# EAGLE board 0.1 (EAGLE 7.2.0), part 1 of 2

Size 160 x 100 mm. Coordinates in mm from the lower left corner, seen from the top.
Outline: 0,0 160,0 160,100 0,100 0,0
Copper layers (1*16): Top 0.035mm / dielectric 1.5mm / Bottom 0.035mm
Design rules "default": minimum track width 10mil, minimum drill 24mil, track to track 8mil, track to pad 8mil, pad to pad 8mil, via to via 8mil, smd to smd 8mil, copper to edge 40mil, drill to drill 8mil, minimum pad ring 10mil, minimum via ring 8mil, stop-mask expansion 4mil, vias tented up to drill 0mil, thermal gap 10mil

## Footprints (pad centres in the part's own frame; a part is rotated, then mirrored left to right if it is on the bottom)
0207/10 = drill 0.813 octagon: 1 -5.08,0; 2 5.08,0
C050-025X075 = drill 0.813 octagon: 1 -2.54,0; 2 2.54,0
E5-10,5 = drill 1.016 pad 2.54: + -2.54,0 | drill 1.016 pad 2.54 octagon: - 2.54,0
E2,5-5 = drill 0.813 pad 1.6: + -1.27,0 | drill 0.813 pad 1.6 octagon: - 1.27,0
E2,5-6 = drill 0.813 pad 1.6: + -1.27,0 | drill 0.813 pad 1.6 octagon: - 1.27,0
C050-035X075 = drill 0.813 octagon: 1 -2.54,0; 2 2.54,0
DIL20 = drill 0.813 long: 1 -11.43,-3.81; 2 -8.89,-3.81; 3 -6.35,-3.81; 4 -3.81,-3.81; 5 -1.27,-3.81; 6 1.27,-3.81; 7 3.81,-3.81; 8 6.35,-3.81; 9 8.89,-3.81; 10 11.43,-3.81; 11 11.43,3.81; 12 8.89,3.81; 13 6.35,3.81; 14 3.81,3.81; 15 1.27,3.81; 16 -1.27,3.81; 17 -3.81,3.81; 18 -6.35,3.81; 19 -8.89,3.81; 20 -11.43,3.81
DIL14 = drill 0.813 long: 1 -7.62,-3.81; 2 -5.08,-3.81; 3 -2.54,-3.81; 4 0,-3.81; 5 2.54,-3.81; 6 5.08,-3.81; 7 7.62,-3.81; 8 7.62,3.81; 9 5.08,3.81; 10 2.54,3.81; 11 0,3.81; 12 -2.54,3.81; 13 -5.08,3.81; 14 -7.62,3.81
DIL08 = drill 0.813 long: 1 -3.81,-3.81; 2 -1.27,-3.81; 3 1.27,-3.81; 4 3.81,-3.81; 5 3.81,3.81; 6 1.27,3.81; 7 -1.27,3.81; 8 -3.81,3.81
DIL24-3 = drill 0.813 long: 1 -13.97,-3.81; 2 -11.43,-3.81; 3 -8.89,-3.81; 4 -6.35,-3.81; 5 -3.81,-3.81; 6 -1.27,-3.81; 7 1.27,-3.81; 8 3.81,-3.81; 9 6.35,-3.81; 10 8.89,-3.81; 11 11.43,-3.81; 12 13.97,-3.81; 13 13.97,3.81; 14 11.43,3.81; 15 8.89,3.81; 16 6.35,3.81; 17 3.81,3.81; 18 1.27,3.81; 19 -1.27,3.81; 20 -3.81,3.81; 21 -6.35,3.81; 22 -8.89,3.81; 23 -11.43,3.81; 24 -13.97,3.81
PICOFUSE = drill 0.813 long: 1 -5.08,0; 2 5.08,0
JP1 = drill 0.914 long: 1 0,-1.27; 2 0,1.27
G2RA = drill 1.321 long: 1 -3.81,-3.683; 2 -3.81,3.81; P 16.18,3.81; S 19.685,-3.683
SFH480 = drill 0.813 long: A 1.27,0; K -1.27,0
P1-20Y = drill 2.007 pad 2.54 long: TP 0,0
TO220H = drill 1.118 long: 1 -2.54,-10.16; 2 0,-10.16; 3 2.54,-10.16 | hole 3.302: 0,4.826
RTRIM64Y = drill 0.61: 1 0,-2.54; 2 -2.54,0; 3 0,2.54
HC49TL-H = drill 0.813: 1 -2.413,-7.62; 2 2.413,-7.62; 3 0,7.874
0617/17 = drill 1.016 octagon: 1 -8.89,0; 2 8.89,0
TO92-CBE = drill 0.813 long: B 0,0; C -2.54,0; E 2.54,0
DO41-10 = drill 1.118: A 5.08,0; C -5.08,0
SOD81 = drill 1.118 long: A 5.08,0; C -5.08,0
DO15-12 = drill 1.118 long: A 6.35,0; C -6.35,0
DO35-10 = drill 0.813 long: A 5.08,0; C -5.08,0
S18P = drill 1.016 long: 1 21.25,0; 2 18.75,0; 3 16.25,0; 4 13.75,0; 5 11.25,0; 6 8.75,0; 7 6.25,0; 8 3.75,0; 9 1.25,0; 10 -1.25,0; 11 -3.75,0; 12 -6.25,0; 13 -8.75,0; 14 -11.25,0; 15 -13.75,0; 16 -16.24,0; 17 -18.755,0; 18 -21.244,0
AK300/2 = drill 1.321 long: 1 -2.515,0; 2 2.489,0
S06P = drill 1.016 long: 1 6.25,0; 2 3.75,0; 3 1.25,0; 4 -1.25,0; 5 -3.75,0; 6 -6.25,0
5566-12 = drill 1.4 square: 1 10.5,-2.75; 2 6.3,-2.75; 3 2.1,-2.75; 4 -2.1,-2.75; 5 -6.3,-2.75; 6 -10.5,-2.75; 7 10.5,2.75; 8 6.3,2.75; 9 2.1,2.75; 10 -2.1,2.75; 11 -6.3,2.75; 12 -10.5,2.75 | hole 3: 15.2,2.29; -15.2,2.29

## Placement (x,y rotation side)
75-  [0207/10]  not placed on the board
C1  [C050-025X075]  0,0 0 top
C1-  [E5-10,5]  0,0 0 top
C2  [E2,5-5]  not placed on the board
C2-  [E5-10,5]  0,0 0 top
C3  [C050-025X075]  not placed on the board
C3-  [E5-10,5]  0,0 0 top
C4  [C050-025X075]  not placed on the board
C4-  [E2,5-6]  0,0 0 top
C5  [C050-025X075]  0,0 0 top
C5-  [E5-10,5]  0,0 0 top
C6  [E2,5-5]  0,0 0 top
C6-  [E5-10,5]  0,0 0 top
C7  [E2,5-6]  0,0 0 top
C8-  [E5-10,5]  0,0 0 top
C9-  330nF  [C050-035X075]  0,0 0 top
C10  [E2,5-5]  0,0 0 top
C10-  330nF  [C050-035X075]  0,0 0 top
C11  [E2,5-5]  0,0 0 top
C11-  [C050-035X075]  not placed on the board
C12  [E2,5-5]  0,0 0 top
C12-  330nF  [C050-035X075]  0,0 0 top
C13  330nF  [C050-035X075]  0,0 0 top
C13-  330nF  [C050-035X075]  0,0 0 top
C14  330nF  [C050-035X075]  0,0 0 top
C14-  [C050-025X075]  not placed on the board
C15  [C050-025X075]  0,0 0 top
C16  [C050-025X075]  0,0 0 top
C16-  [C050-025X075]  0,0 0 top
C17  [C050-025X075]  0,0 0 top
C18  [C050-025X075]  0,0 0 top
C19  [C050-025X075]  0,0 0 top
C19-  [E2,5-5]  0,0 0 top
C20  330nF  [C050-035X075]  0,0 0 top
C22-  [C050-025X075]  0,0 0 top
C23  [C050-025X075]  not placed on the board
C24-  [E2,5-5]  not placed on the board
C25  [E2,5-5]  not placed on the board
C25-  [C050-025X075]  0,0 0 top
C26  330nF  [C050-035X075]  not placed on the board
C26-  [C050-025X075]  not placed on the board
C27-  [C050-025X075]  0,0 0 top
C28  [C050-035X075]  not placed on the board
C28-  [E2,5-5]  not placed on the board
C29  [E2,5-6]  0,0 0 top
C29-  [E2,5-5]  not placed on the board
C30  330nF  [C050-025X075]  not placed on the board
C30-  330nF  [C050-035X075]  not placed on the board
C31  [E2,5-6]  0,0 0 top
C31-  330nF  [C050-035X075]  not placed on the board
C32  [C050-025X075]  0,0 0 top
C33  [E2,5-6]  0,0 0 top
C34  330nF  [C050-035X075]  0,0 0 top
C35  [C050-025X075]  not placed on the board
C36  [C050-025X075]  not placed on the board
C37  [C050-035X075]  not placed on the board
C40  [C050-025X075]  not placed on the board
C41  [C050-025X075]  not placed on the board
C41-  330nF  [C050-035X075]  0,0 0 top
C42  [E2,5-5]  not placed on the board
C43  [E2,5-5]  not placed on the board
C44  330nF  [C050-035X075]  0,0 0 top
C44-  330nF  [C050-035X075]  0,0 0 top
C49  [C050-025X075]  not placed on the board
C50  [C050-025X075]  not placed on the board
C51  [C050-025X075]  not placed on the board
C52  330nF  [C050-035X075]  not placed on the board
C52-  [C050-025X075]  0,0 0 top
C53  330nF  [C050-035X075]  not placed on the board
C54  [E2,5-5]  not placed on the board
C55  [E2,5-5]  not placed on the board
C56  [C050-025X075]  0,0 0 top
C57  [C050-025X075]  0,0 0 top
C57-  [C050-025X075]  not placed on the board
C58  330nF  [C050-035X075]  0,0 0 top
C59  330nF  [C050-035X075]  not placed on the board
C60  330nF  [C050-035X075]  0,0 0 top
C60-  [C050-035X075]  0,0 0 top
C61  [C050-025X075]  0,0 0 top
C62  [C050-025X075]  0,0 0 top
C63  330nF  [C050-035X075]  not placed on the board
C65  [E2,5-5]  not placed on the board
C66  [E2,5-5]  not placed on the board
C69  [C050-025X075]  not placed on the board
C70  [C050-025X075]  not placed on the board
C71  [C050-025X075]  not placed on the board
C72  [C050-025X075]  not placed on the board
C73  [E2,5-5]  not placed on the board
C74  [E2,5-5]  not placed on the board
C76  [C050-025X075]  not placed on the board
C77  [C050-025X075]  not placed on the board
C79  [C050-025X075]  not placed on the board
C81  [C050-025X075]  not placed on the board
C82  330nF  [C050-025X075]  not placed on the board
C83  [C050-025X075]  not placed on the board
C84  [C050-025X075]  not placed on the board
C85  [C050-025X075]  not placed on the board
C86  [C050-025X075]  not placed on the board
C87  [C050-025X075]  not placed on the board
C88  [C050-025X075]  not placed on the board
C91  [C050-025X075]  not placed on the board
C92  [C050-025X075]  not placed on the board
C93  10nF  [C050-025X075]  not placed on the board
C94  [C050-025X075]  0,0 0 top
C97  [C050-025X075]  not placed on the board
C98  330nF  [C050-025X075]  not placed on the board
C98-  10nF  [C050-025X075]  not placed on the board
C99  [C050-025X075]  not placed on the board
C103-  [E2,5-5]  not placed on the board
C104  [E2,5-5]  not placed on the board
C105  [C050-025X075]  not placed on the board
C106  [C050-025X075]  not placed on the board
C106-  330nF  [C050-035X075]  not placed on the board
C107-  [C050-025X075]  not placed on the board
C109  330nF  [C050-035X075]  not placed on the board
C111  330nF  [C050-035X075]  not placed on the board
C112  330nF  [C050-035X075]  not placed on the board
C113  330nF  [C050-035X075]  not placed on the board
C114  330nF  [C050-035X075]  not placed on the board
C115  330nF  [C050-035X075]  not placed on the board
C116  330nF  [C050-035X075]  not placed on the board
C117  330nF  [C050-035X075]  not placed on the board
C118  330nF  [C050-025X075]  not placed on the board
C119-1  [C050-035X075]  0,0 0 top
C120  330nF  [C050-025X075]  not placed on the board
C123  [C050-025X075]  not placed on the board
C126  330nF  [C050-025X075]  not placed on the board
C128-  [C050-025X075]  0,0 0 top
C129-  [C050-025X075]  0,0 0 top
C130  [C050-025X075]  not placed on the board
D1-  [DIL20]  not placed on the board
D2-  [DIL14]  not placed on the board
D3-  [DIL14]  not placed on the board
D5-1  [DIL14]  not placed on the board
D6  [DIL08]  0,0 0 top
D7  [DIL08]  0,0 0 top
D8-AC-FREQ-VOLTAGE/3.12V-FIXED-VOLTAGE  [DIL08]  0,0 0 top
D9-N12/1-TRIANGE-INTEGRATOR-POS/NEG-BIAS-CURR-SWITCH  [DIL08]  0,0 0 top
D10-AC-BAL-SWITCH  [DIL08]  0,0 0 top
D12-2  [DIL08]  not placed on the board
D14  [DIL08]  0,0 0 top
D15  [DIL14]  0,0 0 top
D16  [DIL14]  0,0 0 top
D17-2  [DIL20]  not placed on the board
D18  [DIL24-3]  not placed on the board
F11  FUSEPICOFUSE  [PICOFUSE]  0,0 0 top
IC1  [DIL14]  0,0 0 top
IC6  [DIL14]  0,0 0 top
IC13-AC-MOSFET-DRIVER-OPEN-COLLECTOR  [DIL14]  0,0 0 top
IC16  [DIL14]  0,0 0 top
JP1  [JP1]  not placed on the board
JP2  [JP1]  not placed on the board
JP3  [JP1]  not placed on the board
JP7  [JP1]  not placed on the board
JP8  [JP1]  not placed on the board
JP10  [JP1]  not placed on the board
JP11  [JP1]  not placed on the board
JP12  [JP1]  not placed on the board
JP13  [JP1]  not placed on the board
JP14  [JP1]  not placed on the board
JP15  [JP1]  not placed on the board
JP17  [JP1]  not placed on the board
K1  G2RA  [G2RA]  not placed on the board
LED1/+5V  [SFH480]  not placed on the board
LED1/+15V  [SFH480]  not placed on the board
LED1/-15V  [SFH480]  not placed on the board
LED1/ACDC  [SFH480]  not placed on the board
LED1/RGLSPR  [SFH480]  not placed on the board
LED1/STRSTP  [SFH480]  not placed on the board
LED2/IGRO  [SFH480]  not placed on the board
LED2/IPRUE  [SFH480]  not placed on the board
LED2/POLARITY  [SFH480]  not placed on the board
LED2/PRUE  [SFH480]  not placed on the board
LED2/PRUN  [SFH480]  not placed on the board
LED2/SEKUE  [SFH480]  not placed on the board
LED2/STOER  [SFH480]  not placed on the board
LED2/TEMP  [SFH480]  not placed on the board
M1  TPPAD1-20Y  [P1-20Y]  0,0 0 top
M2  TPPAD1-20Y  [P1-20Y]  0,0 0 top
M3  TPPAD1-20Y  [P1-20Y]  0,0 0 top
M4  TPPAD1-20Y  [P1-20Y]  0,0 0 top
M5  TPPAD1-20Y  [P1-20Y]  0,0 0 top
M6  TPPAD1-20Y  [P1-20Y]  0,0 0 top
M7  TPPAD1-20Y  [P1-20Y]  0,0 0 top
M8  TPPAD1-20Y  [P1-20Y]  0,0 0 top
M10  TPPAD1-20Y  [P1-20Y]  not placed on the board
M11  TPPAD1-20Y  [P1-20Y]  0,0 0 top
M13  TPPAD1-20Y  [P1-20Y]  not placed on the board
M15  TPPAD1-20Y  [P1-20Y]  not placed on the board
M18  TPPAD1-20Y  [P1-20Y]  not placed on the board
M19  TPPAD1-20Y  [P1-20Y]  not placed on the board
M20  TPPAD1-20Y  [P1-20Y]  not placed on the board
M21  TPPAD1-20Y  [P1-20Y]  not placed on the board
M22-AC-BALANCED-AC-FREQ  TPPAD1-20Y  [P1-20Y]  not placed on the board
MINUSPOL  [SFH480]  not placed on the board
N1  7815-PosReg  [TO220H]  not placed on the board
N2  7805-PosReg  [TO220H]  not placed on the board
N3  7915-NegReg  [TO220H]  not placed on the board
N5-TEMP-SENSOR  [DIL08]  not placed on the board
N6  [DIL08]  not placed on the board
N7-?-?-?-TRIANGLE-INTO-VARIABLE-WIDTH-PULSE-(AC-BAL)  [DIL14]  0,0 0 top
N8  [DIL14]  0,0 0 top
N9  [DIL14]  0,0 0 top
N10  [DIL14]  0,0 0 top
N11/FREQ/FREQ/BAL/FREQ  [DIL14]  0,0 0 top
N12  [DIL14]  0,0 0 top
P1  [RTRIM64Y]  not placed on the board
P3  [RTRIM64Y]  not placed on the board
P4  [RTRIM64Y]  not placed on the board
P5  [RTRIM64Y]  not placed on the board
P7-I-MIN  [RTRIM64Y]  not placed on the board
P8  [RTRIM64Y]  not placed on the board
P8-AC-FREQ-MIN  [RTRIM64Y]  not placed on the board
P10-AC-FREQ  [RTRIM64Y]  not placed on the board
P11  [RTRIM64Y]  not placed on the board
P12-AC-BAL  1k  [RTRIM64Y]  not placed on the board
PLUSPOL  [SFH480]  not placed on the board
Q1  [HC49TL-H]  not placed on the board
R1  [0207/10]  not placed on the board
R2  [0207/10]  not placed on the board
R2-  [0207/10]  not placed on the board
R3  [0207/10]  not placed on the board
R4  [0207/10]  0,0 0 top
R4-  22k  [0207/10]  not placed on the board
R5  [0207/10]  0,0 0 top
R5-  [0207/10]  not placed on the board
R6-  [0207/10]  0,0 0 top
R7-  [0207/10]  not placed on the board
R9-  [0207/10]  not placed on the board
R10-  [0207/10]  not placed on the board
R14-  [0207/10]  0,0 0 top
R15-  [0207/10]  0,0 0 top
R16-  [0207/10]  0,0 0 top
R17-  [0207/10]  not placed on the board
R18-  [0207/10]  not placed on the board
R19  [RTRIM64Y]  not placed on the board
R19-  [0207/10]  not placed on the board
R21-  [0207/10]  0,0 0 top
R22-  [0207/10]  0,0 0 top
R23-  [0207/10]  0,0 0 top
R24-  [0207/10]  0,0 0 top
R26-  [0207/10]  not placed on the board
R28  [0207/10]  not placed on the board
R28-  [0207/10]  0,0 0 top
R29  1k  [0207/10]  0,0 0 top
R30  [0207/10]  0,0 0 top
R33-  [0207/10]  0,0 0 top
R34  [0207/10]  0,0 0 top
R35-  [0207/10]  not placed on the board
R37  [0207/10]  not placed on the board
R37-  [0207/10]  not placed on the board
R38  [0207/10]  not placed on the board
R38-  [0207/10]  0,0 0 top
R39  [0207/10]  not placed on the board
R39-  100  [0207/10]  0,0 0 top
R40  [0207/10]  not placed on the board
R43  [0207/10]  0,0 0 top
R44  [0207/10]  0,0 0 top
R44-  [0207/10]  0,0 0 top
R45  [0207/10]  0,0 0 top
R46  [0207/10]  0,0 0 top
R46-  [0207/10]  0,0 0 top
R49  [0207/10]  0,0 0 top
R50  [0207/10]  0,0 0 top
R50-  22k  [0207/10]  0,0 0 top
R51  [0207/10]  0,0 0 top
R51-  [0207/10]  not placed on the board
R52  [0207/10]  0,0 0 top
R52-  [0207/10]  not placed on the board
R53  [0207/10]  0,0 0 top
R53-  [0207/10]  not placed on the board
R54  [0207/10]  0,0 0 top
R54-  [0207/10]  not placed on the board
R55  [0207/10]  not placed on the board
R56  [0207/10]  not placed on the board
R56-  [0207/10]  0,0 0 top
R57-  [0207/10]  0,0 0 top
R58  [0207/10]  not placed on the board
R59  1k  [0207/10]  0,0 0 top
R60  1k  [0207/10]  0,0 0 top
R60-FAT  [0617/17]  not placed on the board
R61-FAT  [0617/17]  not placed on the board
R61-PULLDOWN-GND  10k  [0207/10]  0,0 0 top
R62  22k  [0207/10]  0,0 0 top
R62-FAT  [0617/17]  0,0 0 top
R63  1k  [0207/10]  0,0 0 top
R63-FAT  [0617/17]  0,0 0 top
R64  [0207/10]  not placed on the board
R65-  470  [0207/10]  not placed on the board
R65-+5V-PULLUP  [0207/10]  0,0 0 top
R66  [0207/10]  0,0 0 top
R66-  3,3k  [0207/10]  not placed on the board
R67  [0207/10]  0,0 0 top
R68  [0207/10]  0,0 0 top
R68-  3,3k  [0207/10]  not placed on the board
R69  [0207/10]  0,0 0 top
R69-  [0207/10]  0,0 0 top
R70  [0207/10]  0,0 0 top
R71  4.7k  [0207/10]  not placed on the board
R71-  [0207/10]  0,0 0 top
R72  [0207/10]  not placed on the board
R72-  [0207/10]  0,0 0 top
R73  [0207/10]  not placed on the board
R73-  [0207/10]  not placed on the board
R74  [0207/10]  not placed on the board
R74-  [0207/10]  not placed on the board
R75  [0207/10]  0,0 0 top
R76  [0207/10]  0,0 0 top
R77  [0207/10]  0,0 0 top
R78  [0207/10]  0,0 0 top
R79  [0207/10]  0,0 0 top
R80  [0207/10]  0,0 0 top
R81-  [0207/10]  0,0 0 top
R82-FAT  [0617/17]  0,0 0 top
R83  [0207/10]  0,0 0 top
R83-FAT  [0617/17]  0,0 0 top
R84  [0207/10]  0,0 0 top
R84-FAT  [0617/17]  0,0 0 top
R85-FAT  [0617/17]  0,0 0 top
R86-  [0207/10]  not placed on the board
R87  4.7k  [0207/10]  not placed on the board
R87-  [0207/10]  not placed on the board
R88  22k  [0207/10]  not placed on the board
R89  [0207/10]  not placed on the board
R90-  [0207/10]  not placed on the board
R91  [0207/10]  not placed on the board
R92-  [0207/10]  not placed on the board
R93  [0207/10]  not placed on the board
R94  [0207/10]  not placed on the board
R95  [0207/10]  not placed on the board
R95-  [0207/10]  not placed on the board
R96  [0207/10]  not placed on the board
R96-  [0207/10]  not placed on the board
R97  [0207/10]  not placed on the board
R97-  22k  [0207/10]  not placed on the board
R98  22k  [0207/10]  not placed on the board
R98-  22k  [0207/10]  not placed on the board
R99  [0207/10]  not placed on the board
R99-  22k  [0207/10]  not placed on the board
R100  [0207/10]  not placed on the board
R100-  [0207/10]  not placed on the board
R101  [0207/10]  not placed on the board
R102  [0207/10]  not placed on the board
R102-  [0207/10]  not placed on the board
R103  [0207/10]  not placed on the board
R103-  [0207/10]  not placed on the board
R104  [0207/10]  not placed on the board
R104-  [0207/10]  not placed on the board
R105  22k  [0207/10]  not placed on the board
R105-  [0207/10]  not placed on the board
R106  22k  [0207/10]  not placed on the board
R107  [0207/10]  not placed on the board
R108  22k  [0207/10]  not placed on the board
R108-  [0207/10]  not placed on the board
R109  [0207/10]  not placed on the board
R110  [0207/10]  not placed on the board
R110-  [0207/10]  not placed on the board
R111  [0207/10]  not placed on the board
R112  [0207/10]  not placed on the board
R113  22k  [0207/10]  not placed on the board
R113-  [0207/10]  not placed on the board
R114  [0207/10]  not placed on the board
R116  [0207/10]  not placed on the board
R117-FUSE+15V  FUSEPICOFUSE  [PICOFUSE]  0,0 0 top
R118-FUSE  FUSEPICOFUSE  [PICOFUSE]  0,0 0 top
R119  [0207/10]  not placed on the board
R119-FUSE-  FUSEPICOFUSE  [PICOFUSE]  0,0 0 top
R120  [0207/10]  not placed on the board
R121  [0207/10]  not placed on the board
R122  [0207/10]  not placed on the board
R123  [0207/10]  not placed on the board
R123-  [0207/10]  not placed on the board
R124-  [0207/10]  not placed on the board
R125  [0207/10]  not placed on the board
R127  [0207/10]  not placed on the board
R128  4.7k  [0207/10]  not placed on the board
R129  [0207/10]  not placed on the board
R135-  [0207/10]  not placed on the board
R136-  [0207/10]  not placed on the board
R137-  [0207/10]  not placed on the board
R138-  [0207/10]  not placed on the board
R139-  [0207/10]  not placed on the board
R141-  [0207/10]  not placed on the board
R142  [0207/10]  not placed on the board
R143  [0207/10]  not placed on the board
R144  [0207/10]  not placed on the board
R145  [0207/10]  not placed on the board
R147  [0207/10]  not placed on the board
R148-  [0207/10]  not placed on the board
R149-  [0207/10]  not placed on the board
R150  10k  [0207/10]  0,0 0 top
R150-  [0207/10]  not placed on the board
R151  [0207/10]  not placed on the board
R151-  [0207/10]  not placed on the board
R153-  [0207/10]  0,0 0 top
R154-  [0207/10]  not placed on the board
R155  [0207/10]  not placed on the board
R155-  22k  [0207/10]  not placed on the board
R156  470  [0207/10]  not placed on the board
R156-  [0207/10]  not placed on the board
R157  470  [0207/10]  not placed on the board
R157-  [0207/10]  0,0 0 top
R159  22k  [0207/10]  0,0 0 top
R160  [0207/10]  0,0 0 top
R161  [0207/10]  0,0 0 top
R162  [0207/10]  0,0 0 top
R164-FUSE  FUSEPICOFUSE  [PICOFUSE]  0,0 0 top
R165  [0207/10]  0,0 0 top
R166-  [0207/10]  not placed on the board
R167-  [0207/10]  not placed on the board
R168-  [0207/10]  not placed on the board
R170  [0207/10]  not placed on the board
R171  [0207/10]  not placed on the board
R172  [0207/10]  not placed on the board
R173  22k  [0207/10]  not placed on the board
R174  [0207/10]  not placed on the board
R175  [0207/10]  not placed on the board
R175-  [0207/10]  not placed on the board
R176  [0207/10]  not placed on the board
R177  22k  [0207/10]  not placed on the board
R178  22k  [0207/10]  not placed on the board
R179  [0207/10]  not placed on the board
R180  [0207/10]  not placed on the board
R181  [0207/10]  not placed on the board
R181-  1k  [0207/10]  not placed on the board
R182  [0207/10]  not placed on the board
R183  [0207/10]  not placed on the board
R183-  4.7k  [0207/10]  not placed on the board
R184  [0207/10]  not placed on the board
R184-  4.7k  [0207/10]  not placed on the board
R185  [0207/10]  not placed on the board
R185-  4.7k  [0207/10]  not placed on the board
R186-  4.7k  [0207/10]  not placed on the board
R187-  [0207/10]  not placed on the board
R188  [0207/10]  not placed on the board
R189  [0207/10]  not placed on the board
R190  22k  [0207/10]  not placed on the board
R191  22k  [0207/10]  not placed on the board
R192  22k  [0207/10]  not placed on the board
R193-FEEDBK-2  3,3k  [0207/10]  not placed on the board
R194-FEEDBK-1  4.7k  [0207/10]  not placed on the board
R195  [0207/10]  not placed on the board
R196  [0207/10]  not placed on the board
R197  [0207/10]  not placed on the board
R199  [0207/10]  not placed on the board
R200  [0207/10]  not placed on the board
R201  22k  [0207/10]  not placed on the board
R202  [0207/10]  not placed on the board
R203  22k  [0207/10]  not placed on the board
R208  [0207/10]  not placed on the board
R209  [0207/10]  not placed on the board
R211  22k  [0207/10]  not placed on the board
R212  22k  [0207/10]  not placed on the board
R213-5V-PULLUP  22k  [0207/10]  not placed on the board
R214  22k  [0207/10]  not placed on the board
R220  [0207/10]  not placed on the board
R222  [0207/10]  not placed on the board
R223  22k  [0207/10]  not placed on the board
R226  [0207/10]  not placed on the board
R227  [0207/10]  not placed on the board
R228  4.7k  [0207/10]  not placed on the board
R229  [0207/10]  0,0 0 top
R230  4.7k  [0207/10]  not placed on the board
R232  4.7k  [0207/10]  not placed on the board
R234  4.7k  [0207/10]  not placed on the board
R235  [0207/10]  not placed on the board
R236  [0207/10]  not placed on the board
R237  4.7k  [0207/10]  not placed on the board
R249  [0207/10]  not placed on the board
R250  [0207/10]  not placed on the board
R251  [0207/10]  not placed on the board
R253  [0207/10]  not placed on the board
R254  [0207/10]  not placed on the board
R255  [0207/10]  not placed on the board
R256  [0207/10]  not placed on the board
R257  [0207/10]  not placed on the board
R259  10k  [0207/10]  not placed on the board
R260  10k  [0207/10]  not placed on the board
R261  10k  [0207/10]  not placed on the board
R262  4.7k  [0207/10]  not placed on the board
R263-FUSE  FUSEPICOFUSE  [PICOFUSE]  0,0 0 top
R263-FUSE1  FUSEPICOFUSE  [PICOFUSE]  0,0 0 top
R263-FUSE2+15V  FUSEPICOFUSE  [PICOFUSE]  0,0 0 top
R264  [0207/10]  0,0 0 top
R265  [0207/10]  not placed on the board
R268  [0207/10]  not placed on the board
R269  [0207/10]  not placed on the board
R270  [0207/10]  not placed on the board
R272-FUSE  FUSEPICOFUSE  [PICOFUSE]  0,0 0 top
R273-FUSE  FUSEPICOFUSE  [PICOFUSE]  0,0 0 top
R274-FUSE  FUSEPICOFUSE  [PICOFUSE]  0,0 0 top
R275-FUSE  FUSEPICOFUSE  [PICOFUSE]  0,0 0 top
R276-FUSE  FUSEPICOFUSE  [PICOFUSE]  0,0 0 top
R277  [0207/10]  0,0 0 top
R279  [0207/10]  not placed on the board
R284  [0207/10]  not placed on the board
S2  [JP1]  not placed on the board
S9  [JP1]  not placed on the board
S12-AC-WAVEFORM-SHAPE/RISETIME-1  [JP1]  not placed on the board
S12-AC-WAVEFORM-SHAPE/RISETIME-2  [JP1]  not placed on the board
S22  [JP1]  not placed on the board
S23  [JP1]  not placed on the board
T3  [TO92-CBE]  not placed on the board
T4  [TO92-CBE]  not placed on the board
T5  [TO92-CBE]  not placed on the board
T6  [TO92-CBE]  not placed on the board
T7  [TO92-CBE]  not placed on the board
T8  [TO92-CBE]  not placed on the board
T9  [TO92-CBE]  not placed on the board
T10  [TO92-CBE]  not placed on the board
T11  [TO92-CBE]  not placed on the board
T12  [TO92-CBE]  not placed on the board
T13  [TO92-CBE]  not placed on the board
T14  [TO92-CBE]  not placed on the board
T15  [TO92-CBE]  not placed on the board
T17  [TO92-CBE]  not placed on the board
T18  [TO92-CBE]  not placed on the board
T19  [TO92-CBE]  not placed on the board
T20  [TO92-CBE]  not placed on the board
T21  [TO92-CBE]  not placed on the board
T22  [TO92-CBE]  not placed on the board
T23  [TO92-CBE]  not placed on the board
T24  [TO92-CBE]  not placed on the board
T25  [TO92-CBE]  not placed on the board
TP1  TPPAD1-20Y  [P1-20Y]  0,0 0 top
V1  1N4004  [DO41-10]  0,0 0 top
V1-  1N4004  [DO41-10]  0,0 0 top
V2  BZD23  [SOD81]  0,0 0 top
V3  1N4004  [DO41-10]  0,0 0 top
V4  Diode-0.6V  [DO15-12]  0,0 0 top
V5  Diode-0.6V  [DO15-12]  0,0 0 top
V6  Diode-0.6V  [DO15-12]  0,0 0 top
V6-  BZD23  [SOD81]  0,0 0 top
V7  Diode-0.6V  [DO15-12]  0,0 0 top
V7-  BZD23  [SOD81]  0,0 0 top
V8  1N4148  [DO35-10]  0,0 0 top
V9  1N4148  [DO35-10]  0,0 0 top
V10  1N4148  [DO35-10]  not placed on the board
V11  1N4148  [DO35-10]  not placed on the board
V12  1N4148  [DO35-10]  not placed on the board
V13  1N4004  [DO41-10]  0,0 0 top
V14  Z-4.7V  [SOD81]  0,0 0 top
V17  1N4148  [DO35-10]  not placed on the board
V18  1N4148  [DO35-10]  not placed on the board
V19  1N4148  [DO35-10]  not placed on the board
V20  1N4148  [DO35-10]  not placed on the board
V21  1N4148  [DO35-10]  not placed on the board
V22  1N4148  [DO35-10]  not placed on the board
V22-NO-ZENER?  BZD23  [SOD81]  not placed on the board
V23  1N4148  [DO35-10]  not placed on the board
V24  Diode-0.6V  [DO15-12]  0,0 0 top
V25  BZD23  [SOD81]  not placed on the board
V26  1N4148  [DO35-10]  not placed on the board
V26-  1N4148  [DO35-10]  not placed on the board
V27  1N4148  [DO35-10]  not placed on the board
V28  1N4148  [DO35-10]  not placed on the board
V29  1N4148  [DO35-10]  not placed on the board
V30  1N4148  [DO35-10]  not placed on the board
V30-NOZENER  BZD23  [SOD81]  0,0 0 top
V31  1N4004  [DO41-10]  not placed on the board
V32  Diode-0.6V  [DO15-12]  0,0 0 top
V34  1N4148  [DO35-10]  not placed on the board
V35  1N4148  [DO35-10]  not placed on the board
V37  BZD23  [SOD81]  not placed on the board
V38  1N4004  [DO41-10]  not placed on the board
V39  1N4004  [DO41-10]  not placed on the board
V41  1N4148  [DO35-10]  0,0 0 top
V42  1N4148  [DO35-10]  0,0 0 top
V42-  1N4148  [DO35-10]  0,0 0 top
V43  1N4148  [DO35-10]  0,0 0 top
V43-  1N4148  [DO35-10]  0,0 0 top
V44  Diode-0.6V  [DO15-12]  0,0 0 top
V45  1N4148  [DO35-10]  not placed on the board
V46  1N4148  [DO35-10]  not placed on the board
V47  1N4148  [DO35-10]  not placed on the board
V48  1N4148  [DO35-10]  not placed on the board
V49  1N4004  [DO41-10]  0,0 0 top
V50  1N4004  [DO41-10]  0,0 0 top
V51  1N4148  [DO35-10]  not placed on the board
V52  1N4148  [DO35-10]  not placed on the board
V53  1N4148  [DO35-10]  not placed on the board
V54  1N4148  [DO35-10]  not placed on the board
V55  1N4148  [DO35-10]  not placed on the board
V55-  1N4148  [DO35-10]  not placed on the board
V56  1N4148  [DO35-10]  not placed on the board
V57  1N4148  [DO35-10]  not placed on the board
V58  1N4004  [DO41-10]  0,0 0 top
V61  Z-2.2V  [SOD81]  not placed on the board
V62  1N4148  [DO35-10]  0,0 0 top
V65  1N4148  [DO35-10]  not placed on the board
V66  1N4148  [DO35-10]  0,0 0 top
V66-NOZENER  BZD23  [SOD81]  not placed on the board
V67  1N4148  [DO35-10]  not placed on the board
V70  Diode-0.6V  [DO15-12]  not placed on the board
V72  Diode-0.6V  [DO15-12]  not placed on the board
V73  Diode-0.6V  [DO15-12]  not placed on the board
V74  Diode-0.6V  [DO15-12]  not placed on the board
V75  Diode-0.6V  [DO15-12]  not placed on the board
V76  Diode-0.6V  [DO15-12]  not placed on the board
V77  Diode-0.6V  [DO15-12]  not placed on the board
V78  Diode-0.6V  [DO15-12]  not placed on the board
V79  Diode-0.6V  [DO15-12]  not placed on the board
V80  Diode-0.6V  [DO15-12]  not placed on the board
V81  Diode-0.6V  [DO15-12]  not placed on the board
V82-NOZENER  BZD23  [SOD81]  0,0 0 top
V83  Diode-0.6V  [DO15-12]  not placed on the board
V84  1N4148  [DO35-10]  not placed on the board
V85  1N4148  [DO35-10]  not placed on the board
V91  1N4148  [DO35-10]  not placed on the board
V92  1N4148  [DO35-10]  not placed on the board
V93  1N4148  [DO35-10]  not placed on the board
V97-NOZENER  BZD23  [SOD81]  0,0 0 top
V100-NOZENER  BZD23  [SOD81]  not placed on the board
V101  1N4004  [DO41-10]  not placed on the board
V102  1N4148  [DO35-10]  not placed on the board
V102-NOZENER  BZD23  [SOD81]  0,0 0 top
V104  1N4148  [DO35-10]  not placed on the board
V105  1N4148  [DO35-10]  not placed on the board
V109-NOZENER  BZD23  [SOD81]  not placed on the board
V110  BZD23  [SOD81]  0,0 0 top
V113-NOZENER  BZD23  [SOD81]  0,0 0 top
V114  Diode-0.6V  [DO15-12]  not placed on the board
V115  1N4148  [DO35-10]  0,0 0 top
V120  1N4004  [DO41-10]  not placed on the board
V121  1N4004  [DO41-10]  not placed on the board
X1  [S18P]  not placed on the board
X2  [S18P]  not placed on the board
X3  [AK300/2]  not placed on the board
X4-  [AK300/2]  not placed on the board
X5  [S06P]  not placed on the board
X6  5566-12  [5566-12]  0,0 0 top
X7-  [AK300/2]  not placed on the board
X8  [AK300/2]  not placed on the board
X9  [S06P]  not placed on the board
X10  [S06P]  not placed on the board
X11  [S06P]  not placed on the board
X12  [AK300/2]  not placed on the board
X13  [AK300/2]  not placed on the board

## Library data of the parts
75- C1-C6 C9- C10 C10- C11 C11- C12 C12- C13 C13- C14 C14- C15 C16 C16- C17-C19 C19- C20 C22- C23 C24- C25 C25- C26 C26- C27- C28 C28- C29- C30 C30- C31- C32 C34-C37 C40 C41 C41- C42-C44 C44- C49-C52 C52- C53-C57 C57- C58-C60 C60- C61-C63 C65 C66 C69-C74 C76 C77 C79 C81-C88 C91-C94 C97 C98 C98- C99 C103- C104-C106 C106- C107- C109 C111-C118 C119-1 C120 C123 C126 C128- C129- C130 P1 P3-P5 P7-I-MIN P8 P8-AC-FREQ-MIN P10-AC-FREQ P11 P12-AC-BAL R1 R2 R2- R3 R4 R4- R5 R5- R6- R7- R9- R10- R14- R15- R16- R17- R18- R19 R19- R21- R22- R23- R24- R26- R28 R28- R29 R30 R33- R34 R35- R37 R37- R38 R38- R39 R39- R40 R43 R44 R44- R45 R46 R46- R49 R50 R50- R51 R51- R52 R52- R53 R53- R54 R54- R55 R56 R56- R57- R58-R60 R60-FAT R61-FAT R61-PULLDOWN-GND R62 R62-FAT R63 R63-FAT R64 R65- R65-+5V-PULLUP R66 R66- R67 R68 R68- R69 R69- R70 R71 R71- R72 R72- R73 R73- R74 R74- R75-R80 R81- R82-FAT R83 R83-FAT R84 R84-FAT R85-FAT R86- R87 R87- R88 R89 R90- R91 R92- R93-R95 R95- R96 R96- R97 R97- R98 R98- R99 R99- R100 R100- R101 R102 R102- R103 R103- R104 R104- R105 R105- R106-R108 R108- R109 R110 R110- R111-R113 R113- R114 R116 R119-R123 R123- R124- R125 R127-R129 R135- R136- R137- R138- R139- R141- R142-R145 R147 R148- R149- R150 R150- R151 R151- R153- R154- R155 R155- R156 R156- R157 R157- R159-R162 R165 R166- R167- R168- R170-R175 R175- R176-R181 R181- R182 R183 R183- R184 R184- R185 R185- R186- R187- R188-R192 R193-FEEDBK-2 R194-FEEDBK-1 R195-R197 R199-R203 R208 R209 R211 R212 R213-5V-PULLUP R214 R220 R222 R223 R226-R230 R232 R234-R237 R249-R251 R253-R257 R259-R262 R264 R265 R268-R270 R277 R279 R284 = resistor
C1- C2- C3- C4- C5- C6- C7 C8- C29 C31 C33 = rcl
D1- D2- D3- D5-1 D12-2 D17-2 D18 N5-TEMP-SENSOR N6 = ic-package
D6 D7 D8-AC-FREQ-VOLTAGE/3.12V-FIXED-VOLTAGE D9-N12/1-TRIANGE-INTEGRATOR-POS/NEG-BIAS-CURR-SWITCH D10-AC-BAL-SWITCH D14-D16 IC6 IC13-AC-MOSFET-DRIVER-OPEN-COLLECTOR IC16 N7-?-?-?-TRIANGLE-INTO-VARIABLE-WIDTH-PULSE-(AC-BAL) N8-N10 N11/FREQ/FREQ/BAL/FREQ N12 = 11-Wig-parts-1
F11 R117-FUSE+15V R118-FUSE R119-FUSE- R164-FUSE R263-FUSE R263-FUSE1 R263-FUSE2+15V R272-FUSE R273-FUSE R274-FUSE R275-FUSE R276-FUSE = fuse; OC_FARNELL: unknown; OC_NEWARK: unknown
IC1 = 11-Wig-parts-good
JP1-JP3 JP7 JP8 JP10-JP15 JP17 S2 S9 S12-AC-WAVEFORM-SHAPE/RISETIME-1 S12-AC-WAVEFORM-SHAPE/RISETIME-2 S22 S23 = jumper
K1 = relay; OC_FARNELL: unknown; OC_NEWARK: unknown
LED1/+5V LED1/+15V LED1/-15V LED1/ACDC LED1/RGLSPR LED1/STRSTP LED2/IGRO LED2/IPRUE LED2/POLARITY LED2/PRUE LED2/PRUN LED2/SEKUE LED2/STOER LED2/TEMP MINUSPOL PLUSPOL = led
M1-M8 M10 M11 M13 M15 M18-M21 M22-AC-BALANCED-AC-FREQ TP1 = testpad
N1-N3 = linear
Q1 = crystal; OC_FARNELL: unknown; OC_NEWARK: unknown
T3-T7 T17-T20 = transistor-neu-to92
T8-T15 T21-T25 = transistor
V1 V1- V2-V6 V6- V7 V7- V8-V14 V17-V22 V22-NO-ZENER? V23-V26 V26- V27-V30 V30-NOZENER V31 V32 V34 V35 V37-V39 V41 V42 V42- V43 V43- V44-V55 V55- V56-V58 V61 V62 V65 V66 V66-NOZENER V67 V70 V72-V81 V82-NOZENER V83-V85 V91-V93 V97-NOZENER V100-NOZENER V101 V102 V102-NOZENER V104 V105 V109-NOZENER V110 V113-NOZENER V114 V115 V120 V121 = diode
X1 X2 X5 X9-X11 = con-amp-mt; OC_FARNELL: unknown; OC_NEWARK: unknown
X3 X4- X7- X8 X12 X13 = con-ptr500; OC_FARNELL: unknown; OC_NEWARK: unknown
X6 = con-molex; OC_FARNELL: unknown; OC_NEWARK: unknown

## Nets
3.12V-FIXED: D8-AC-FREQ-VOLTAGE/3.12V-FIXED-VOLTAGE.7 R188.2 R189.1
4X-TEMPSWITCHES-COMBINED: C12.+ IC1.13 R1.2 R63.1
+5VDC: C5-.+ C6-.+ C98.1 C120.1 D15.14 D16.14 D17-2.20 D18.24 IC1.14 IC13-AC-MOSFET-DRIVER-OPEN-COLLECTOR.14 N2.3 R2-.2 R65-+5V-PULLUP.2 R212.1 R213-5V-PULLUP.1 R214.1 R253.2 R254.2 R255.2 R256.2 R279.1 R284.1
+5VDC-IN: C4-.+ N2.1 X5.3
+15VDC: C10.+ C11-.2 C28-.+ C37.1 C43.+ C54.+ C73.+ C103-.+ C104.+ D6.8 D7.3 D7.8 D8-AC-FREQ-VOLTAGE/3.12V-FIXED-VOLTAGE.3 D8-AC-FREQ-VOLTAGE/3.12V-FIXED-VOLTAGE.8 D9-N12/1-TRIANGE-INTEGRATOR-POS/NEG-BIAS-CURR-SWITCH.3 D9-N12/1-TRIANGE-INTEGRATOR-POS/NEG-BIAS-CURR-SWITCH.8 D10-AC-BAL-SWITCH.3 D10-AC-BAL-SWITCH.8 D14.8 IC6.11 JP1.1 N5-TEMP-SENSOR.7 N7-?-?-?-TRIANGLE-INTO-VARIABLE-WIDTH-PULSE-(AC-BAL).11 N8.11 N9.3 N10.3 N11/FREQ/FREQ/BAL/FREQ.11 N12.11 R40.1 R52-.1 R56.1 R93.1 R94.2 R102.2 R103-.1 R103.2 R106.1 R107.1 R108-.1 R108.1 R109.1 R112.2 R119.2 R123.2 R128.2 R166-.1 R167-.1 R182.1 R188.1 R211.1 R236.2 R249.2 R250.2 R260.1 R261.1 R263-FUSE2+15V.1 S9.2 T3.E T4.E T5.E T6.E T7.E V9.C V13.A V18.C V20.C V25.C V34.C V38.C V45.C V47.C V51.C V55-.C V55.C V58.A V105.C X1.5 X1.18 X2.2 X2.9 X6.2 X10.3 X11.3
+15VDC-IN: C1-.+ N1.1 X5.1
+15VDC-PSU: C2-.+ C3-.+ C60-.2 D12-2.8 N1.3 R117-FUSE+15V.2 R263-FUSE2+15V.2
+33VDC-IN: R50-.2 X5.6
-15VDC: C8-.- C11.- C24-.- C29-.- C55.- C66.+ C74.- D6.5 D7.5 D8-AC-FREQ-VOLTAGE/3.12V-FIXED-VOLTAGE.5 D9-N12/1-TRIANGE-INTEGRATOR-POS/NEG-BIAS-CURR-SWITCH.5 D10-AC-BAL-SWITCH.5 D14.5 IC6.7 LED1/-15V.K N3.3 N5-TEMP-SENSOR.4 N7-?-?-?-TRIANGLE-INTO-VARIABLE-WIDTH-PULSE-(AC-BAL).7 N8.7 N11/FREQ/FREQ/BAL/FREQ.7 N12.7 R116.2 R183-.1 V1.A V8.A V19.A V35.A V52.A V54.A V56.A V76.A X1.7 X2.7
-15VDC-IN: C7.- N3.2 X5.2
??12: R202.2 V61.A
AC-BAL-VOLTAGE-1: N11/FREQ/FREQ/BAL/FREQ.8 N11/FREQ/FREQ/BAL/FREQ.10 P12-AC-BAL.1
AC-BAL-VOLTAGE-2: P12-AC-BAL.2 R184-.1
AC-BAL-VOLTAGE-INVERTED: D10-AC-BAL-SWITCH.7 M18.TP N12.10 R194-FEEDBK-1.2
AC-BAL-VOLTAGE-INVERTED-TRIANGLE-TRIGGER-VOLTS: C26.1 N7-?-?-?-TRIANGLE-INTO-VARIABLE-WIDTH-PULSE-(AC-BAL).14 R100.2
AC-BALANCE/0V=20%EP: R178.2 X9.2
AC-BALANCED-AC-FREQ-PULSES-1: N7-?-?-?-TRIANGLE-INTO-VARIABLE-WIDTH-PULSE-(AC-BAL).12 R127.2 V30.C
AC-BALANCED-AC-FREQ-PULSES-2: R101.2 V30.A
AC-BALANCED-AC-FREQ-PULSES-3: JP15.2 M22-AC-BALANCED-AC-FREQ.TP R101.1 V37.C
AC-BALANCED-AC-FREQ-PULSES-4: C84.1 D18.4 JP8.1 JP15.1 R214.2
AC-FREQ-TRIANGLE-1: C41.2 M20.TP N12.3 R113.2 R208.1 R209.2
AC-FREQ-TRIANGLE-2: N7-?-?-?-TRIANGLE-INTO-VARIABLE-WIDTH-PULSE-(AC-BAL).13 R113.1 R127.1
AC-FREQ-VADJ-3: P8-AC-FREQ-MIN.2 R196.1
AC-FREQ-VOLTAGE-2: C52-.1 N8.3 R4-.1 R100-.2 S12-AC-WAVEFORM-SHAPE/RISETIME-1.2
AC-FREQ-VOLTAGE-ADJUSTED: D8-AC-FREQ-VOLTAGE/3.12V-FIXED-VOLTAGE.6 M19.TP N11/FREQ/FREQ/BAL/FREQ.4 N11/FREQ/FREQ/BAL/FREQ.6
AC-FREQ-VOLTAGE-BUFFERED: N11/FREQ/FREQ/BAL/FREQ.1 N11/FREQ/FREQ/BAL/FREQ.3 P10-AC-FREQ.3
AC-FREQ-VOLTAGE-BUFFERED-ADJ-1: P10-AC-FREQ.2 R195.2
AC-FREQ-VOLTAGE-BUFFERED-ADJ-2: C71.1 N11/FREQ/FREQ/BAL/FREQ.5 R195.1 R196.2
AC-FREQ-VOLTAGE-IN: C69.1 N11/FREQ/FREQ/BAL/FREQ.2 R177.1 V45.A V46.C
AC-FREQ-VOLTS/3.12V-FIXED: C72.2 D8-AC-FREQ-VOLTAGE/3.12V-FIXED-VOLTAGE.4 R187-.1 R190.1
AC-FREQ-VOLTS/3.12V-FIXED-2: N11/FREQ/FREQ/BAL/FREQ.14 R190.2 R191.1
AC-FREQ/0V=50HZ: R177.2 X9.1
AC-NEG-RAMP-CURRENT: D9-N12/1-TRIANGE-INTEGRATOR-POS/NEG-BIAS-CURR-SWITCH.7 R187-.2
AC-POS-RAMP-CURRENT: D9-N12/1-TRIANGE-INTEGRATOR-POS/NEG-BIAS-CURR-SWITCH.6 R197.2
AC-SQUAREWAVE-(FROM-AC-TRIANGLE)=>TRIANGLE-INTEGRATOR-BIAS-SWITCH&MINUS-LED: C42.- M21.TP MINUSPOL.A N12.4 R71.1 V10.C V11.A
AC/DC-AC=15V: R222.1 R226.2 S9.1 X9.4
ALL-TEMPSWITCHES-COMBINED: R1.1 V28.C V29.C V92.C V93.C
CHOPPER-AC-FREQ: D9-N12/1-TRIANGE-INTEGRATOR-POS/NEG-BIAS-CURR-SWITCH.2 R71.2 T5.C V12.C
D6-D7-SWITCH-ENABLE: D6.2 D7.2 D16.13 R58.1 V82-NOZENER.C V113-NOZENER.C
D6-D7-SWITCH-ENABLE-1: IC1.10 V113-NOZENER.A
D6-D7-SWITCH-ENABLE-2: IC1.4 V82-NOZENER.A
D8-SWITCH-ENABLE-(FIXED/VARIABLE-AC-FREQ): D8-AC-FREQ-VOLTAGE/3.12V-FIXED-VOLTAGE.2 M6.TP N10.2 R112.1 R202.1 V100-NOZENER.C V102-NOZENER.C
D8-SWITCH-ENABLE-(FIXED/VARIABLE-AC-FREQ)-FROM-X1/2&X3/2: C40.2 N10.5 R161.2 R162.2
GND [GND]: C1-.- C1.2 C2-.- C3-.- C4-.- C5.2 C6.- C7.+ C8-.+ C10.- C11-.1 C11.+ C12.- C13.1 C14-.2 C14.1 C15.2 C16.2 C17.2 C18.2 C19.2 C20.1 C23.1 C24-.+ C25.- C26-.1 C26.2 C27-.1 C28-.- C28.2 C29-.+ C29.+ C30-.2 C30.2 C31-.2 C31.- C33.- C34.2 C35.2 C36.1 C37.2 C40.1 C41-.1 C42.+ C43.- C44-.1 C44.2 C49.2 C50.1 C52.2 C53.2 C54.- C55.+ C56.1 C57-.2 C57.1 C59.1 C60-.1 C60.2 C61.1 C62.1 C65.+ C66.- C69.2 C70.1 C71.2 C72.1 C76.1 C77.1 C79.1 C81.2 C82.2 C83.2 C84.2 C85.2 C86.2 C87.2 C88.1 C91.1 C92.1 C93.1 C94.2 C97.1 C98-.1 C98.2 C99.1 C103-.- C104.- C105.2 C106.2 C107-.2 C111.1 C112.1 C113.1 C114.1 C115.1 C116.1 C117.1 C118.1 C120.2 C123.1 C126.1 C128-.2 C129-.2 C130.1 D1-.1 D1-.20 D2-.7 D2-.11 D2-.13 D3-.11 D5-1.7 D6.1 D7.1 D8-AC-FREQ-VOLTAGE/3.12V-FIXED-VOLTAGE.1 D9-N12/1-TRIANGE-INTEGRATOR-POS/NEG-BIAS-CURR-SWITCH.1 D10-AC-BAL-SWITCH.1 D12-2.1 D14.1 D15.7 D16.7 D17-2.10 D18.9 D18.10 D18.12 IC1.7 IC13-AC-MOSFET-DRIVER-OPEN-COLLECTOR.7 IC16.7 K1.1 LED1/+5V.K LED1/+15V.K LED1/ACDC.K LED1/RGLSPR.K LED1/STRSTP.K N1.2 N2.2 N3.1 N6.1 N6.4 N9.12 N10.12 P7-I-MIN.3 P8-AC-FREQ-MIN.3 P8.3 R3.1 R17-.1 R19.2 R19.3 R26-.1 R30.2 R39.1 R44-.1 R44.2 R51-.1 R54-.1 R58.2 R60-FAT.1 R61-FAT.1 R61-PULLDOWN-GND.1 R62-FAT.1 R63-FAT.1 R63.2 R64.2 R67.1 R70.2 R78.2 R79.2 R80.1 R83.2 R84.2 R87.2 R97-.1 R97.2 R104.2 R105.1 R110.1 R122.2 R124-.1 R137-.2 R138-.1 R139-.1 R143.1 R145.1 R149-.2 R156-.2 R157.2 R165.1 R170.1 R171.1 R172.1 R173.1 R174.1 R179.2 R180.2 R181-.1 R181.2 R183.1 R184.1 R185.1 R186-.1 R189.2 R192.2 R199.1 R251.1 R259.1 R265.2 R269.1 T8.C T9.C T10.C T11.C T12.C T13.B T14.B T15.C T17.C T18.C T19.C T20.C T25.C V1.C V5.A V12.A V13.C V24.A V32.A V37.A V39.A V44.A V46.A V50.A V57.A V70.A V72.A V73.A V74.A V75.A V76.C V77.A V78.A V79.A V80.A V81.A V83.A V85.C V104.A V114.A V120.A X1.4 X1.6 X1.11 X1.13 X1.16 X2.8 X5.4 X5.5 X6.3 X10.2 X11.2
I-PULS: R200.2 X9.3
INP-1/1-AC-SWITCH-DELAY?: C81.1 C99.2 D17-2.1 D18.1 N10.14 R65-+5V-PULLUP.1
INP-1/7-: C87.1 D17-2.2 D18.7 IC1.8 V115.A
INP-4/X-TEMP-SWITCHES: C30.1 D17-2.4 IC1.12
INP-5/X-: C105.1 D17-2.5 R253.1 V102-NOZENER.A
INP-6/X-: C106.1 D17-2.6 N9.2 R147.2 R255.1
INP-7/X-: C107-.1 D17-2.7 R256.1 V91.A
INP-8/X-: C106-.2 D17-2.8 R254.1
INP-11/X-: C109.1 D17-2.11 R2.1 R257.1 V66-NOZENER.C
INP-X/2-N5-TEMP-SENSOR-(0=>GOOD): C83.1 C119-1.1 D16.9 D18.2 M13.TP N9.14 R212.2 R277.1
INP-X/3-FIXED/VARIABLE-AC-FREQ: C82.1 D18.3 R213-5V-PULLUP.2 V100-NOZENER.A
INP-X/5-: C85.1 D18.5
INP-X/6-PLUS-MINUS-NOT-D6-D7-SWITCH-ENABLE-1: C86.1 D18.6 IC1.6 IC1.11
INP-X/15-FROM-OUTP-X/22: C98-.2 D18.14 R59.1
INP-X/23-FROM-OUTP-X/15: C93.2 D18.23 R60.1
INV-AC-FREQ-VOLTS/-3.12V-FIXED: N11/FREQ/FREQ/BAL/FREQ.12 R191.2 R197.1
N5-NEG-INP: C22-.2 N5-TEMP-SENSOR.2 R66-.1 R69-.1
N5-POS-INP: N5-TEMP-SENSOR.3 R68-.1
N5-TEMP-OUT: N5-TEMP-SENSOR.6 R39-.2 R72-.2 R155.2
N5-TEMP-OUT-2: C36.2 R110-.2 R155.1
N5-TEMP-OUT-3: N9.9 R110-.1 R270.2
N9-8-FIXED-VOLTAGE-LEVEL: C119-1.2 N9.8 R29.1 R108-.2
N10-P4/+2.411VDC-FIXED: N10.4 R102.1 R103.1 R104.1
N10-P9-FIXED-VOLTAGE-AC-SWITCH-DELAY?: N10.9 R105.2 R106.2
N10-P11-FIXED-VOLTAGE: N10.11 R108.2 R110.2
N12-P2-TO-GND: N12.2 R269.2
N12-P5-TO-GND: N12.5 R199.2
N12-P9-TO-GND: N12.9 R186-.2
N12-P13-FIXED-VOLTAGE: N12.13 R259.2 R260.2
N$1: R153-.2 R270.1
N$2: LED2/POLARITY.K R268.2
N$4: R175-.2 X2.12
N$5: N8.5 V20.A V21.C
N$6: C14.2 R75.2 R76.2
N$7: LED2/IGRO.A LED2/IPRUE.A LED2/POLARITY.A LED2/PRUE.A LED2/PRUN.A LED2/SEKUE.A LED2/STOER.A LED2/TEMP.A
N$8: D16.10 V114.C X6.6
N$9: R175-.1 V55.A V56.C
N$12: N6.8 R55.1 V49.C V121.C X12.1 X13.1
N$13: N7-?-?-?-TRIANGLE-INTO-VARIABLE-WIDTH-PULSE-(AC-BAL).10 R111.1 R141-.1
N$14: C28.1 N12.14 R261.2 R262.2 V104.C V105.A
N$17: C1.1 N7-?-?-?-TRIANGLE-INTO-VARIABLE-WIDTH-PULSE-(AC-BAL).9 R135-.1 R136-.2 R137-.1 V48.C V55-.A
N$18: T11.E V49.A V50.C X13.2
N$19: IC1.2 JP8.2
N$20: LED2/IGRO.K R228.2
N$21: JP2.2 JP3.2 R235.2
N$22: LED2/PRUN.K R232.2
N$23: LED2/SEKUE.K R237.2
N$24: LED2/TEMP.K R234.2
N$25: C32.2 V5.C X4-.2
N$26: LED1/RGLSPR.A R154-.1
N$27: MINUSPOL.K PLUSPOL.A R265.1
N$28: T12.E V120.C V121.A X12.2
N$29: D15.8 R232.1 V75.C X2.3
N$30: D15.12 JP3.1 R234.1 V77.C X2.1
N$33: C70.2 N11/FREQ/FREQ/BAL/FREQ.9 R178.1 V47.A V57.C
N$34: T7.C V7.A
N$35: R105-.2 R251.2
N$36: R193-FEEDBK-2.1 R194-FEEDBK-1.1
N$37: C15.1 N6.3 R69.2
N$38: IC6.8 IC6.10 R91.2 V18.A V19.C
N$39: C31-.1 R68.2 V41.C
N$45: N12.8 R184-.2 R185-.2 R193-FEEDBK-2.2
N$50: C52-.2 N8.1 R98-.2 R99-.2 R100-.1
N$51: M15.TP T8.E
N$52: N10.13 R68.1 R109.2
N$53: R203.2 V53.C
N$54: R141-.2 V27.A
N$55: C63.2 N8.13 R166-.2 R167-.2 R168-.2
N$56: C63.1 R95-.1 R168-.1 R257.2 V66-NOZENER.A
N$57: M1.TP N8.10 R35-.1 R151-.1
N$58: N8.8 R38.2 R150-.1
N$59: N8.12 N8.14 R176.1 V38.A V39.C
N$66: JP10.2 JP11.2 JP12.2 JP13.2 R73-.1 R90-.2
N$67: V3.A X1.17
N$70: JP7.1 N7-?-?-?-TRIANGLE-INTO-VARIABLE-WIDTH-PULSE-(AC-BAL).8 R111.2 R139-.2
N$72: D7.6 P8.2
N$74: D10-AC-BAL-SWITCH.4 R100.1
N$75: R28.1 V26.A
N$78: D1-.8 R53.1 R54.1
N$79: JP7.2 R138-.2
N$81: N7-?-?-?-TRIANGLE-INTO-VARIABLE-WIDTH-PULSE-(AC-BAL).5 R124-.2
N$84: R129.1 V26-.A V26.C V27.C
N$86: LED1/+5V.A R2-.1
N$89: N7-?-?-?-TRIANGLE-INTO-VARIABLE-WIDTH-PULSE-(AC-BAL).1 R96.1 R113-.2 R114.1 V23.A
N$90: N7-?-?-?-TRIANGLE-INTO-VARIABLE-WIDTH-PULSE-(AC-BAL).2 R97.1
N$91: C4.2 M2.TP N7-?-?-?-TRIANGLE-INTO-VARIABLE-WIDTH-PULSE-(AC-BAL).3 V23.C V26-.C
N$92: N7-?-?-?-TRIANGLE-INTO-VARIABLE-WIDTH-PULSE-(AC-BAL).4 V17.C V22.C
N$93: R98.1 V91.C
N$94: R98.2 R99.2 T9.B
N$95: D10-AC-BAL-SWITCH.6 R99.1
N$96: C3.2 R28.2 R128.1 V17.A
N$97: P8.1 R94.1
N$98: N8.6 P5.1
N$100: P4.3 R95-.2
N$101: N8.4 P4.1
N$102: D6.7 P4.2
N$103: P5.3 R96-.2
N$104: D6.6 P5.2
N$105: N8.2 R97-.2
N$106: C59.2 R155-.2 V102.A
N$111: R121.1 R122.1
N$114: R116.1 R120.1
N$116: C106-.1 C109.2
N$117: JP10.1 R174.2
N$122: N8.9 R37.2 R148-.2
N$127: C129-.1 D14.2 R38-.2 V110.A
N$130: R150-.2 R151-.2
N$133: D1-.2 R180.1
N$134: R29.2 R30.1
N$135: R19.1 R151.2
N$136: R82-FAT.1 R83-FAT.1
N$137: M4.TP R69.1 R84-FAT.1 R85-FAT.1 X1.14
N$138: R82-FAT.2 R83-FAT.2 R84-FAT.2 R85-FAT.2
N$139: S22.1 X1.9
N$140: S23.1 X1.8
N$141: T6.C V66.A
N$142: D1-.3 R55.2 R181.1
N$144: C5.1 D1-.14 P1.3
N$145: D1-.15 R84.1
N$146: C16.1 D1-.17 R79.1
N$147: IC16.8 R14-.2
N$148: D1-.19 R77.1
N$149: C18.1 D1-.13 R75.1 R76.1 R78.1
N$151: C17.1 D1-.16 R70.1 V43.C
N$152: IC16.6 R15-.2
N$153: D5-1.14 R14-.1 R15-.1
N$154: D5-1.3 R16-.1
N$155: D5-1.4 R21-.1
N$156: R28-.1 R38-.1 R56.2 T15.E V7-.C V110.C
N$157: D2-.14 D3-.14 IC16.14
N$158: R250.1 V93.A X11.1
N$160: D5-1.9 R22-.2
N$161: D5-1.10 R23-.2
N$165: R262.1 X10.6 X11.6
N$166: C22-.1 S2.1
N$167: D6.4 R98-.1
N$168: R249.1 V92.A X10.1
N$171: D15.2 JP2.1 R228.1 V72.C X2.6
N$177: N9.11 R9-.2 R19-.1 R151.1
N$182: N9.13 R9-.1
N$184: C27-.2 R39-.1
N$185: R71-.1 R72-.1
N$186: R69-.2 R71-.2
N$187: R264.2 V6.C V7.C
N$188: V4.A V6.A
N$189: D12-2.3 R150.1
N$190: R150.2 V42-.C
N$192: D12-2.7 R159.1 R160.1
N$193: R157-.2 R160.2
N$197: R161.1 V43-.C
N$198: 75-.2 JP11.1 R173.2
N$199: JP12.1 R170.2 R171.2 R172.2 R175.1
N$203: IC6.2 R86-.2
N$204: IC6.4 R5-.2 V6-.C V109-NOZENER.A
N$205: IC6.5 R37-.1
N$206: IC6.6 R4-.2 R5-.1
N$207: C25-.2 D14.4 IC6.14 R7-.2 R18-.1
N$208: C25-.1 IC6.12 R37-.2 S12-AC-WAVEFORM-SHAPE/RISETIME-2.2
N$209: IC6.9 R90-.1
N$210: IC6.13 R26-.2
N$211: R153-.1 R277.2
N$212: R7-.1 V109-NOZENER.C
N$213: R157-.1 T7.B V42-.A
N$214: C62.2 D12-2.2 D12-2.6 R159.2
N$215: C61.2 D12-2.5
N$217: C5-.- C6-.-
N$218: R162.1 R165.2 V4.C V43-.A X1.2 X3.2
N$219: R264.1 X1.1 X3.1
N$221: C94.1 R60-FAT.2 R61-FAT.2 R62-FAT.2 R63-FAT.2 R156.2 X1.3
N$224: R201.1 T3.C V14.A
N$225: C79.2 R200.1 R201.2
N$226: D7.4 R99-.1
N$227: R211.2 T5.B V14.C
N$228: R203.1 T3.B V61.C
N$229: R236.1 T4.B V84.A
N$230: D6.3 R279.2 V79.C X6.1
N$231: K1.2 T4.C V85.A
N$232: K1.P X8.1
N$233: K1.S X8.2
N$234: C73.- C74.+
N$235: C2.- C51.2 R96-.1 V21.A V48.A
N$236: R155-.1 V31.C V115.C
N$237: V101.C X6.11
N$238: R88.1 R89.2 X6.10
N$239: R135-.2 X6.9
N$240: D16.8 V81.C X6.8
N$241: D16.6 V80.C X6.7
N$242: D16.2 V78.C X6.12
N$243: D16.12 V83.C X6.5
N$244: C50.2 M11.TP R91.1 X2.11 X6.4
N$245: C23.2 R87-.2 X2.10
N$246: V74.C X2.4
N$247: D16.5 R284.2
N$250: IC6.1 IC6.3 R87-.1 V34.A V35.C
N$251: C65.-
N$252: R92-.2 X2.13
N$253: R136-.1 X2.14
N$254: C2.+ R176.2 X2.15
N$255: C51.1 R92-.1
N$256: JP1.2 R154-.2 V31.A X2.17
N$257: LED1/+15V.A R40.2
N$258: R62.1 R227.2 V65.C
N$259: P11.3 R3.2
N$260: P11.1 R183-.2
N$261: P11.2 R185-.1
N$262: R73.2 R74.2
N$264: R72.2 V10.A
N$265: R74.1 V11.C
N$268: R38.1 V52.C
N$270: M8.TP R125.2 S12-AC-WAVEFORM-SHAPE/RISETIME-1.1 S12-AC-WAVEFORM-SHAPE/RISETIME-2.1
N$273: C3.1 R95.2
N$274: N7-?-?-?-TRIANGLE-INTO-VARIABLE-WIDTH-PULSE-(AC-BAL).6 R95.1 R123-.2 R125.1 V22.A
N$275: C4.1 R96.2
N$277: P7-I-MIN.1 R93.2
N$278: D7.7 P7-I-MIN.2
N$280: C25.+ N10.8 R107.2 T9.E V25.A
N$281: R235.1 V84.C
N$282: V65.A X2.18
N$283: LED1/-15V.A R39.2
N$284: LED1/ACDC.A R226.1
N$285: LED1/STRSTP.A R227.1
N$286: C26-.2 R35-.2
N$288: R148-.1 R149-.1
N$289: R156-.1 T8.B V102.C
N$291: R37.1 R145.2 V54.C
N$292: R142.2 R143.2 V51.A
N$295: R68-.2 R156.1 V8.C V9.A
N$296: R104-.2 R123-.1
N$297: R144.2 V53.A
N$298: N9.4 P3.2 P3.3 R17-.2
N$299: R144.1 S23.2
N$300: R142.1 S22.2
N$301: R66.1 V2.C V3.C
N$302: C14-.1 N9.5 N9.10 R50-.1 R51-.2 R147.1
N$303: V2.A V66.C
N$304: C57-.1 N9.7 R102-.1 R104-.1 R105-.1 TP1.TP
N$305: M5.TP R53-.2
N$306: N9.6 R103-.2 T14.C T14.E
N$307: R10-.2 R19-.2 R52-.2 T13.C
N$308: C128-.1 D14.3 R28-.2 V7-.A
N$309: P3.1 R10-.1
N$310: R102-.2 V22-NO-ZENER?.C
N$311: R18-.2 V6-.A
N$312: R53-.1 R54-.2 T13.E
N$313: M3.TP R129.2
N$314: C123.2 V30-NOZENER.A V62.A
N$316: R67.2 T11.B V42.A
N$317: JP13.1 M10.TP R73-.2 R74-.2 R86-.1 R113-.1 R175.2
N$318: C30-.1 R66.2 V42.C
N$320: C35.1 N9.1 R4.1 V22-NO-ZENER?.A V43.A
N$323: JP17.1 V97-NOZENER.A
N$325: R45.1 T15.B V62.C
N$326: R44.1 R45.2
N$334: R220.1 T6.B V67.A
N$335: R65-.2 R157.1
N$336: R65-.1 R66-.2
N$337: R229.1 V67.C
N$338: R229.2 V101.A
N$340: R89.1 R220.2
N$341: 75-.1 R74-.1
N$342: C49.1 IC1.1 R88.2 R183.2
N$344: C126.2 IC1.9 R61-PULLDOWN-GND.2 R62.2
N$346: R4.2 V58.C
N$347: R83.1 T12.B V41.A
N$348: R6-.1 R43.2
N$349: D14.7 R43.1
N$350: D14.6 R6-.2
N$351: R56-.1 R57-.1
N$353: R46-.1 V97-NOZENER.C
N$354: R44-.2 R46-.2 T25.B
N$356: C20.2 D1-.11 R56-.2 R57-.2
N$357: C58.2
N$358: C19.1 R5.2
N$360: N6.2 R80.2 R81-.1
N$361: P1.1 P1.2 R51.2 R52.2
N$362: R50.1 R51.1 R52.1
N$363: D2-.6 D2-.9 R46.2
N$364: C44.1 D1-.10 R50.2
N$365: C56.2 D1-.9
N$366: C57.2 D1-.7
N$367: C58.1 D1-.6
N$368: C13.2 C29.- C44-.2 C60.1 D1-.4 D1-.5
N$369: T17.E T21.C V24.C X7-.1
N$370: C16-.1 V44.C X7-.2
N$371: R22-.1 T18.B T22.B
N$372: C6.+ C41-.2 R33-.1 R34.2
N$373: C33.+ T21.E T22.E T23.E T24.E
N$374: R23-.1 T17.B T21.B
N$375: N6.7 R81-.2
N$376: R21-.2 T19.B T23.B
N$377: C32.1 T20.E T24.C
N$378: R33-.2 T25.E
N$379: T19.E T23.C V32.C X4-.1
N$382: R16-.2 T20.B T24.B
N$385: C16-.2 T18.E T22.C
NEG-2.5V-REFERENCE-VOLTAGE: R120.2 R121.2 T10.E
NOT-NOT-D6-D7-SWITCH-ENABLE-1: C52.1 IC1.3 R184.2 R222.2
OUTP-12/X-TEMP-LED: C116.2 D15.13 D17-2.12
OUTP-13/X-SEKUE-LED: C117.2 D17-2.13 IC13-AC-MOSFET-DRIVER-OPEN-COLLECTOR.13
OUTP-14/X-UNUSED?: C115.2 D15.11 D17-2.14 N10.10 R64.1
OUTP-15/X-PRUN-LED: C114.2 C130.2 D15.9 D17-2.15
OUTP-16/X-UNUSED?: C113.2 D15.5 D17-2.16 JP14.2
OUTP-17/X-STOER-LED: C112.2 D15.3 D16.3 D17-2.17
OUTP-18/X-D10-VARIABLE/FIXED-AC-BAL/IGRO-LED: C111.2 D10-AC-BAL-SWITCH.2 D15.1 D16.1 D17-2.18 JP17.2
OUTP-19/INP-8: C88.2 C118.2 D17-2.19 D18.8
OUTP-X/15-TO-INP-X/23: D18.15 R60.2
OUTP-X/16-POLARITY: C97.2 D18.16 IC13-AC-MOSFET-DRIVER-OPEN-COLLECTOR.11
OUTP-X/17-OUTP-X/18-X11-POS-OPC-X10-NEG-OPC: C77.2 D18.17 IC13-AC-MOSFET-DRIVER-OPEN-COLLECTOR.5 IC13-AC-MOSFET-DRIVER-OPEN-COLLECTOR.9
OUTP-X/18-X10-POS-OPC-X11-NEG-OPC: C76.2 D16.11 D18.18 IC13-AC-MOSFET-DRIVER-OPEN-COLLECTOR.1 IC13-AC-MOSFET-DRIVER-OPEN-COLLECTOR.3
OUTP-X/19-UNUSED?-ALWAYS=1: C92.2 D18.19 R87.1
OUTP-X/20: C91.2 D18.20 R5.1 R34.1
OUTP-X/21-D14-ENABLE-LOGIC: D18.21 V30-NOZENER.C
OUTP-X/22-TO-INP-X/14: D18.22 R59.2
P8-P1=>+15V: P8-AC-FREQ-MIN.1 R182.2
P10-P1=>GND: P10-AC-FREQ.1 R179.1
PLUS/MINUS-1: R223.1 X9.5
PLUS/MINUS-2: C53.1 IC1.5 R185.2 R223.2
POLAR: IC13-AC-MOSFET-DRIVER-OPEN-COLLECTOR.10 R268.1 V70.C X9.6
REF-VNEG: R114.2 T10.B
SEKUE-LED-DRIVE: IC13-AC-MOSFET-DRIVER-OPEN-COLLECTOR.12 R237.1
STOERUNG-LED: LED2/STOER.K R230.2
STOERUNG-LED-DRIVE-OUT: D15.4 R230.1 V73.C X2.5
TO-GND-R-1: P12-AC-BAL.3 R181-.2
TO-GND-R-192: N11/FREQ/FREQ/BAL/FREQ.13 R192.1
TO-INP-11/X-: N12.12 R2.2
TRIANGLE-INPUT=>SQUAREWAVE: N12.6 R72.1 R73.1 R208.2
TRIANGLE-INTEGRATOR-VARIABLE-BIAS-CURRENT-(AC-FREQ): C41.1 D9-N12/1-TRIANGE-INTEGRATOR-POS/NEG-BIAS-CURR-SWITCH.4 N12.1 R209.1
X1-TEMPSWITCH-1: R123.1 V29.A X1.10
X1-TEMPSWITCH-2: R119.1 V28.A X1.12
X10-4-OPTOCOUPL-POS: IC13-AC-MOSFET-DRIVER-OPEN-COLLECTOR.2 X10.4
X10-5-OPTOCOUPL-NEG: IC13-AC-MOSFET-DRIVER-OPEN-COLLECTOR.8 X10.5
X11-4-OPTOCOUPL-POS: IC13-AC-MOSFET-DRIVER-OPEN-COLLECTOR.6 X11.4
X11-5-OPTOCOUPL-NEG: IC13-AC-MOSFET-DRIVER-OPEN-COLLECTOR.4 X11.5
